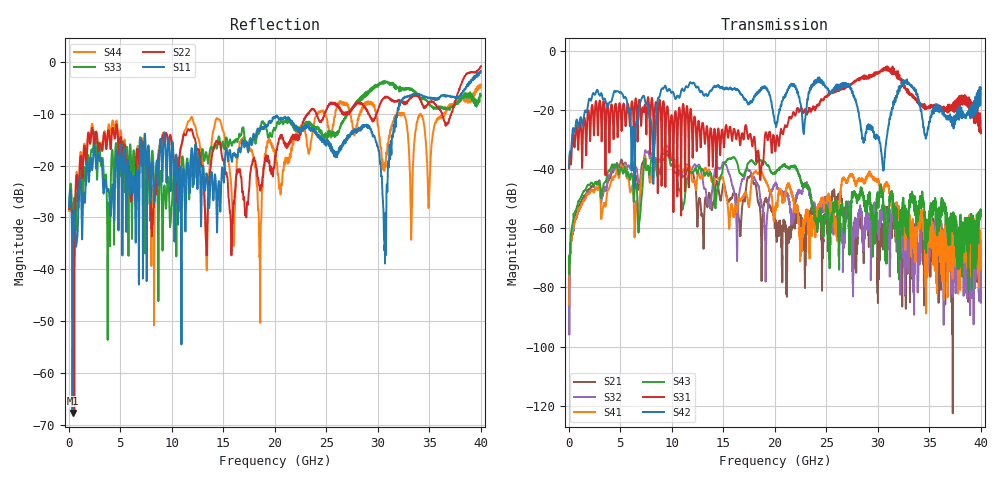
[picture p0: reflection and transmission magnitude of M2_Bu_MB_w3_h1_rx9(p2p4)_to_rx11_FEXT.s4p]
! S11 = S11
! S12 = S12
! S13 = S13
! S14 = S14
! S21 = S21
! S22 = S22
! S23 = S23
! S24 = S24
! S31 = S31
! S32 = S32
! S33 = S33
! S34 = S34
! S41 = S41
! S42 = S42
! S43 = S43
! S44 = S44
! FILE: \\englab.brocade.com\shares\Groups\SIT\Work\Shaohua\IEEE_channels\M2_Bu_MB_w3_h1_rx9(p2p4)_to_rx11_FEXT.s4p
!$DUT_CFG_DESC: Default 4-Port Configuration
!$NUMBER_PORTS: 4
!$DIFF_PORT_MAP: 1|2P|2|2P|0|UC|0|UC|
!$PORT_MAP: PNA 1|1|<<<<<<|TS 2|2|>>>>>>|PNA 2|3|<<<<<<|TS 4|4|>>>>>>|
# MHz S RI R 50.00
! FREQ  S11  S12  S13  S14
!  S21  S22  S23  S24
!  S31  S32  S33  S34
!  S41  S42  S43  S44
!  REAL  IMAG  REAL  IMAG  REAL  IMAG  REAL  IMAG
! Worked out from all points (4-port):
!   3996 points, 50 MHz to 40 GHz, reference 50 ohm
!   strongest paths, dB at 50 MHz, 10.04 GHz, 20.03 GHz, 30.02 GHz, 40 GHz:
!     S42: -39.3, -13.9, -24.3, -28.8, -12.3
!     S31: -39.7, -22.5, -33.3, -7.5, -26.9
!     S43: -72.4, -38.2, -41.5, -50.2, -54.3
!     S41: -85.9, -34.8, -53.3, -43.7, -65.3
!     S32: -81.4, -35.1, -45.1, -57.5, -70.6
!     S21: -79.9, -36.5, -56.8, -68.1, -70.4
!   lowest |S11| = -67.7 dB at 380 MHz (marker M1), VSWR 1.00, Z = 50 + j0.0384 ohm
!   |S11| at or under -10 dB: start of sweep to 31.89 GHz
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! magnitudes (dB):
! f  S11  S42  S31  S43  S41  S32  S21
! 50 MHz  -28.0  -39.3  -39.7  -72.4  -85.9  -81.4  -79.9
! 380 MHz  -67.7  -27.1  -28.5  -58.4  -60.9  -61.4  -60.3
! 9.51 GHz  -23.1  -13.0  -19.9  -35.0  -32.2  -32.2  -33.7
! 18.7 GHz  -12.8  -13.1  -39.2  -37.0  -40.8  -51.2  -71.4
! 30.64 GHz  -35.5  -36.6  -6.1  -60.2  -45.7  -56.3  -56.2
! 32.56 GHz  -7.0  -10.1  -12.5  -56.1  -62.1  -65.4  -66.4
! 40 GHz  -1.8  -12.3  -26.9  -54.3  -65.3  -70.6  -70.4
